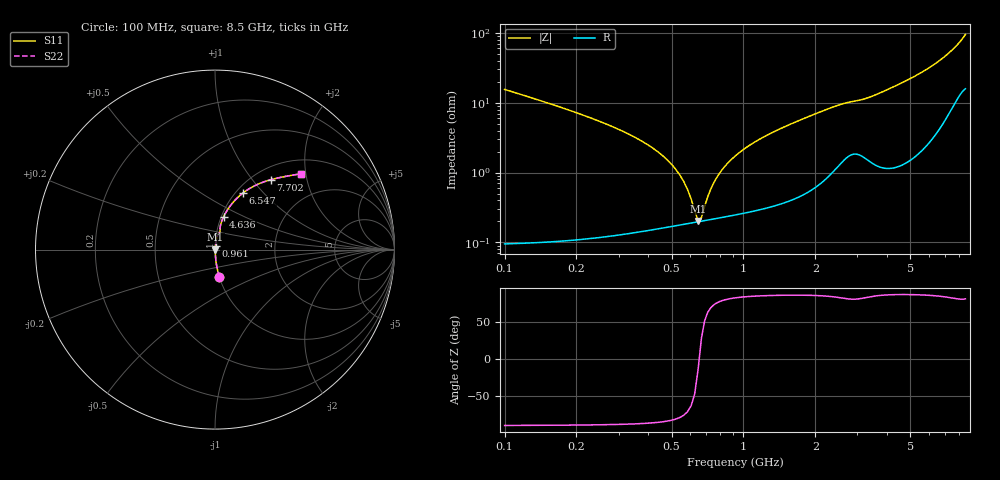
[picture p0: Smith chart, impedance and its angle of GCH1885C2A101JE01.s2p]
!Murata Part Number: GCH1885C2A101JE01
!These Parameters are Measured in Series Mode Connection
!Data Generated on Mar 13, 2026
!  o--ll--o
!Port1  Port2
!  o------o
!Operation Temp=25[degC], DC Bias Voltage=0[V]
!Freq. Start=100[MHz] Stop=9[GHz] 401[Steps]
# Hz S RI R 50
!Freq.(Hz) S11(Real) S11(Imag) S21(Real) S21(Imag) S12(Real) S12(Imag) S22(Real) S22(Imag)
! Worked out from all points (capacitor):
!   401 points, 100 MHz to 8.5 GHz, reference 50 ohm
!   read as one part in series: C = 100 pF near 142 MHz
!   lowest |Z| = 203 mohm at 646 MHz (marker M1)
!   series resonance near 652.8 MHz, so ESL is about 590 pH
!   S11 on the Smith chart (normalised r, x): 100 MHz: 1.00, -0.31; 961 MHz: 1.01, +0.04; 4.636 GHz: 1.03, +0.39; 6.547 GHz: 1.08, +0.78; 7.702 GHz: 1.20, +1.24; 8.5 GHz: 1.32, +1.88
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1e8  0.0244 -0.1514  0.9756 0.1514  0.9756 0.1514  0.0244 -0.1514
2.47e8  0.00417 -0.0547  0.9958 0.0547  0.9958 0.0547  0.00417 -0.0547
4.78e8  0.00187 -0.0152  0.9981 0.0152  0.9981 0.0152  0.00187 -0.0152
5.41e8  0.00185 -0.00908  0.9982 0.00908  0.9982 0.00908  0.00185 -0.00908
6.25e8  0.00193 -0.00209  0.9981 0.00209  0.9981 0.00209  0.00193 -0.00209
6.46e8  0.00197 -0.000498  0.998 0.000498  0.998 0.000498  0.00197 -0.000498
6.88e8  0.00205 0.00253  0.998 -0.00253  0.998 -0.00253  0.00205 0.00253
7.51e8  0.0022 0.00675  0.9978 -0.00675  0.9978 -0.00675  0.0022 0.00675
7.93e8  0.00232 0.0094  0.9977 -0.0094  0.9977 -0.0094  0.00232 0.0094
8.56e8  0.00252 0.0132  0.9975 -0.0132  0.9975 -0.0132  0.00252 0.0132
9.61e8  0.00289 0.019  0.9971 -0.019  0.9971 -0.019  0.00289 0.019
1.192e9  0.00392 0.0308  0.9961 -0.0308  0.9961 -0.0308  0.00392 0.0308
1.507e9  0.00583 0.0456  0.9942 -0.0456  0.9942 -0.0456  0.00583 0.0456
2.242e9  0.0146 0.0786  0.9854 -0.0786  0.9854 -0.0786  0.0146 0.0786
2.914e9  0.0281 0.0989  0.9719 -0.0989  0.9719 -0.0989  0.0281 0.0989
4.3e9  0.0394 0.1634  0.9606 -0.1634  0.9606 -0.1634  0.0394 0.1634
4.636e9  0.0479 0.1831  0.9521 -0.1831  0.9521 -0.1831  0.0479 0.1831
5.707e9  0.0924 0.2533  0.9076 -0.2533  0.9076 -0.2533  0.0924 0.2533
6.547e9  0.1559 0.3153  0.8441 -0.3153  0.8441 -0.3153  0.1559 0.3153
7.114e9  0.221 0.3558  0.779 -0.3558  0.779 -0.3558  0.221 0.3558
7.702e9  0.311 0.3895  0.689 -0.3895  0.689 -0.3895  0.311 0.3895
8.5e9  0.4788 0.4221  0.5212 -0.4221  0.5212 -0.4221  0.4788 0.4221
